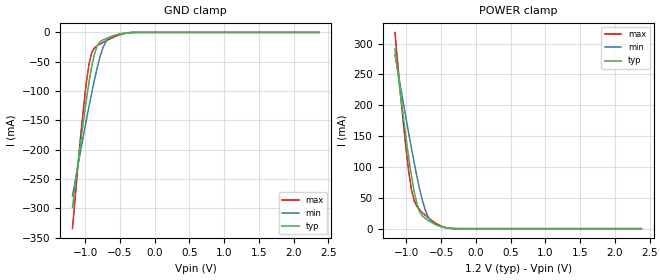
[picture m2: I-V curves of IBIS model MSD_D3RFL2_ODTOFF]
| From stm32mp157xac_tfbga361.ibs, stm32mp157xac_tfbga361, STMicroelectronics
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[Model] MSD_D3RFL2_ODTOFF
Model_type   Input
C_comp 2.255pF   2.172pF   2.373pF
Vinh = 820.000mV
Vinl = 380.000mV
[Model Spec]
Vinh   820.000mV   790.000mV   870.000mV
Vinl   380.000mV   350.000mV   430.000mV
[Temperature Range]   25.000   125.000   -40.000
[Voltage Range]   1.200V   1.140V   1.300V
[GND Clamp Reference]   0.00V   0.00V   0.00V
[POWER Clamp Reference]   1.200V   1.140V   1.300V
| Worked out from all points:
|   GND clamp passes 1 mA (typ) near -0.41 V on its own axis
|   POWER clamp passes 1 mA (typ) near -0.41 V on its own axis
[GND Clamp]
-1.182V   -298.7mA   -278.8mA   -334.6mA
-1.064V   -186.5mA   -201.2mA   -176.5mA
-984.9mV  -117.2mA   -151mA     -87.71mA
-945.5mV  -85.9mA    -126.8mA   -54.95mA
-906.1mV  -58.53mA   -103.4mA   -34.88mA
-866.7mV  -37.07mA   -81.25mA   -26.52mA
-827.3mV  -23.31mA   -60.73mA   -22.77mA
-748.5mV  -13.21mA   -27.8mA    -17.44mA
-709.1mV  -11.06mA   -17.22mA   -14.97mA
-630.3mV  -7.606mA   -7.312mA   -10.35mA
-472.7mV  -2.342mA   -2.056mA   -3.037mA
2.364V    24.05nA    406.6nA    2.603nA
[Power Clamp]
-1.164V   291.7mA    282.1mA    318.2mA
-1.085V   217.9mA    230.4mA    219.1mA
-1.006V   147.8mA    179.6mA    130.3mA
-966.7mV  115.3mA    154.7mA    92.57mA
-927.3mV  85.58mA    130.4mA    63.26mA
-887.9mV  59.89mA    107mA      45.2mA
-809.1mV  27.4mA     63.99mA    30.58mA
-730.3mV  16.7mA     30.88mA    21.97mA
-690.9mV  13.64mA    20.08mA    18.15mA
-572.7mV  6.466mA    6.412mA    8.539mA
-336.4mV  182.5uA    350.9uA    204.7uA
2.382V    -20.25nA   -432nA     -2.13nA
